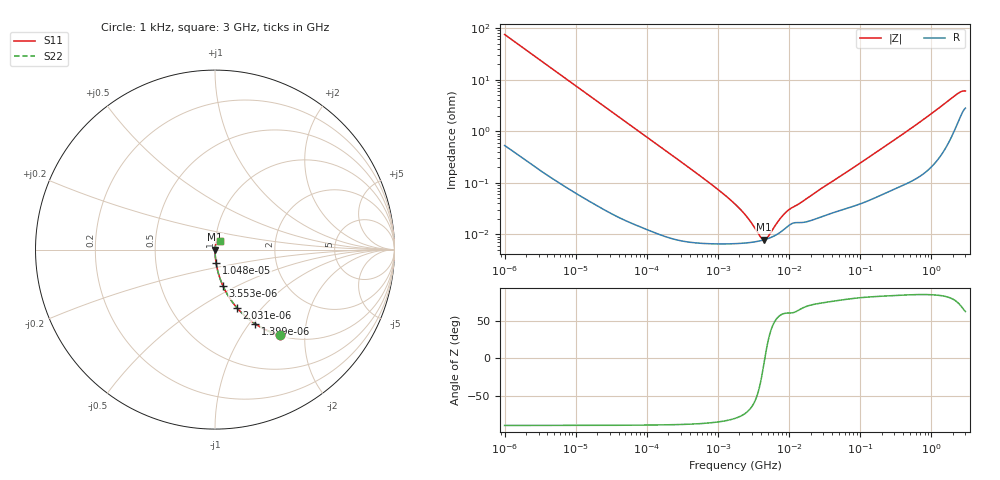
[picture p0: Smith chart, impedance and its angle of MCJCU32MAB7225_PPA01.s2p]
! MCJCU32MAB7225_PPA01  S-PARAMETER MODEL  ( Standard Model )
! Model Generated by TAIYO YUDEN Corporation (http://www.ty-top.com)
! Version 1.0
! TAIYO YUDEN Control No. 220601
! Copyright(c) 2015 TAIYO YUDEN CO.,LTD. All Rights Reserved.
! Product Description (link to TY-COMPAS)
! https://ds.yuden.co.jp/TYCOMPAS/or/detail?pn=MCJCU32MAB7225KPPA01&u=M
! Products Name : Multilayer Ceramic Capacitors
! Characteristics :
!  Capacitance : 2.2 [uF] , Rated Voltage : 50 [V] , TCC : X7R
!  Case Size : 3.2 x 2.5 / 0.126 x 0.098 [mm/inch] , Thickness : 2.5 / 0.098 [mm/inch]
!  (Conditions: Temperature = 25 [degC] , DC Bias Voltage = 0 [V])
! External Node Assignments :
!  1  o---| |---o  2
! GND o---------o GND
! Frequency Range : 1kHz  -  3GHz  [ 401 STEP ]
# MHZ S RI R 50
! Freq[MHz].  S11 Real  S11 Imag  S21 Real  S21 Imag  S12 Real  S12 Imag  S22 Real  S22 Imag
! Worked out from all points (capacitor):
!   401 points, 1 kHz to 3 GHz, reference 50 ohm
!   read as one part in series: C = 2.12 uF near 1.077 kHz
!   lowest |Z| = 7.87 mohm at 4.399 MHz (marker M1)
!   series resonance near 4.551 MHz, so ESL is about 580 pH
!   S11 on the Smith chart (normalised r, x): 1 kHz: 1.01, -1.50; 1.399 kHz: 1.01, -1.07; 2.031 kHz: 1.01, -0.74; 3.553 kHz: 1.00, -0.42; 10.47 kHz: 1.00, -0.14; 3 GHz: 1.06, +0.11
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0.001  0.361 -0.4768  0.639 0.4768  0.639 0.4768  0.361 -0.4768
0.001399  0.2255 -0.4144  0.7745 0.4144  0.7745 0.4144  0.2255 -0.4144
0.002031  0.1225 -0.3243  0.8775 0.3243  0.8775 0.3243  0.1225 -0.3243
0.003553  0.0445 -0.2026  0.9555 0.2026  0.9555 0.2026  0.0445 -0.2026
0.010475  0.0058 -0.0719  0.9942 0.0719  0.9942 0.0719  0.0058 -0.0719
0.01216  0.0044 -0.0621  0.9956 0.0621  0.9956 0.0621  0.0044 -0.0621
0.147855  0.000127 -0.0052  0.9999 0.0052  0.9999 0.0052  0.000127 -0.0052
0.791611  6.64e-05 -0.000946  0.9999 0.000946  0.9999 0.000946  6.64e-05 -0.000946
1.732051  6.6e-05 -0.000381  0.9999 0.000381  0.9999 0.000381  6.6e-05 -0.000381
2.514714  6.82e-05 -0.000213  0.9999 0.000213  0.9999 0.000213  6.82e-05 -0.000213
3.651041  7.33e-05 -7.5e-05  0.9999 7.5e-05  0.9999 7.5e-05  7.33e-05 -7.5e-05
3.93371  7.49e-05 -4.93e-05  0.9999 4.93e-05  0.9999 4.93e-05  7.49e-05 -4.93e-05
4.399271  7.79e-05 -1.14e-05  0.9999 1.14e-05  0.9999 1.14e-05  7.79e-05 -1.14e-05
5.106836  8.32e-05 3.87e-05  0.9999 -3.87e-05  0.9999 -3.87e-05  8.32e-05 3.87e-05
5.502215  8.66e-05 6.39e-05  0.9999 -6.39e-05  0.9999 -6.39e-05  8.66e-05 6.39e-05
7.414467  0.000108 0.000167  0.9999 -0.000167  0.9999 -0.000167  0.000108 0.000167
9.625639  0.000144 0.000253  0.9999 -0.000253  0.9999 -0.000253  0.000144 0.000253
21.06097  0.000189 0.000557  0.9998 -0.000557  0.9998 -0.000557  0.000189 0.000557
256.0921  0.000713 0.00576  0.9993 -0.00576  0.9993 -0.00576  0.000713 0.00576
2226.275  0.0145 0.0482  0.9855 -0.0482  0.9855 -0.0482  0.0145 0.0482
2584.342  0.0223 0.0523  0.9777 -0.0523  0.9777 -0.0523  0.0223 0.0523
3000  0.0298 0.0502  0.9702 -0.0502  0.9702 -0.0502  0.0298 0.0502
